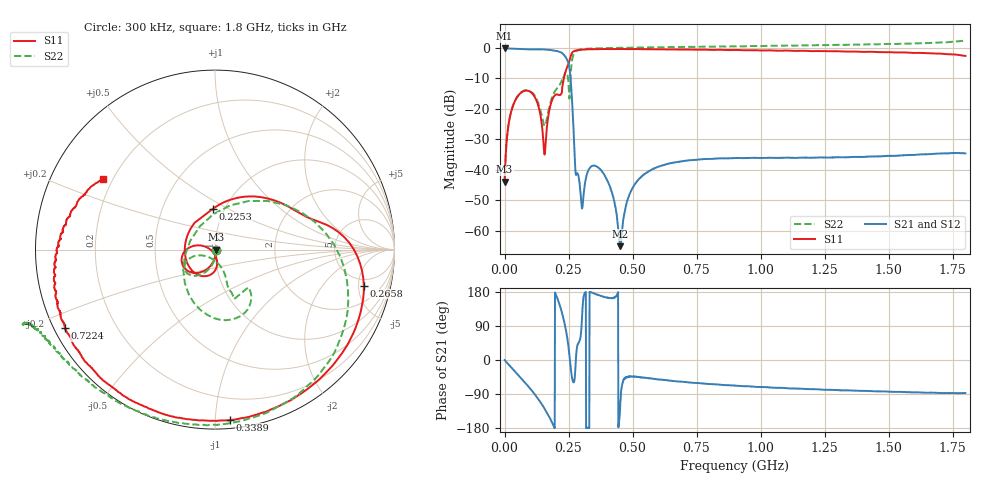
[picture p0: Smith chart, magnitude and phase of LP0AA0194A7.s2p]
!Agilent Technologies,E8358A,US41080443,A.07.50.56
!Agilent E8358A: A.07.50.56
!Date: Wednesday, May 23, 2018 10:03:50
!Correction: S11(Full 2 Port(1,2))
!S21(Full 2 Port(1,2))
!S12(Full 2 Port(1,2))
!S22(Full 2 Port(1,2))
!S2P File: Measurements: S11, S21, S12, S22:
# Hz S  dB  R 50
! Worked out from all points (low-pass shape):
!   1601 points, 300 kHz to 1.8 GHz, reference 50 ohm
!   highest |S21| = -0.11 dB at 300 kHz (marker M1); lowest = -65.0 dB at 451.3 MHz (marker M2)
!   |S21| within 3 dB of the highest: start of sweep to 239.3 MHz
!   lowest |S11| = -43.9 dB at 300 kHz (marker M3), VSWR 1.01, Z = 50.6 - j0.101 ohm
!   |S11| at or under -10 dB: start of sweep to 231.7 MHz
!   |S22| runs from -44.1 to 2.5 dB; largest |S21 - S12| = 0.0093
!   S11 on the Smith chart (normalised r, x): 300 kHz: 1.01, -0.00; 225.3 MHz: 0.88, +0.42; 265.8 MHz: 3.91, -5.78; 338.9 MHz: 0.05, -1.09; 722.4 MHz: 0.03, -0.25; 1.8 GHz: 0.16, +0.28
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300000  -43.86 -8.9  -0.11 -0.2  -0.06 -0.2  -44.08 -9.8
1.8297e7  -23.82 -97.2  -0.19 -13.7  -0.11 -13.7  -23.80 -95.3
4.304288e7  -17.02 -119.6  -0.28 -32.0  -0.21 -32.0  -16.95 -114.5
9.0285e7  -14.05 -157.8  -0.46 -67.6  -0.40 -67.7  -13.84 -144.3
1.296534e8  -18.34 170.1  -0.47 -101.1  -0.40 -101.1  -17.61 -162.3
1.566489e8  -34.98 -132.8  -0.51 -128.6  -0.45 -128.6  -25.58 -117.6
1.971422e8  -15.51 -121.1  -0.90 178.3  -0.84 178.2  -14.19 -70.1
2.252625e8  -12.89 93.4  -1.73 122.5  -1.67 122.5  -11.05 -48.5
2.477588e8  -5.65 22.1  -4.53 45.5  -4.47 45.4  -9.88 -111.2
2.657558e8  -1.38 -13.6  -20.32 -53.2  -20.24 -53.2  -3.09 -3.4
2.792535e8  -0.81 -37.6  -41.68 8.3  -41.62 8.0  -1.05 -43.2
3.006249e8  -0.58 -60.5  -51.49 87.1  -51.57 86.6  -0.47 -69.8
3.388686e8  -0.42 -85.1  -38.85 178.4  -38.81 178.3  -0.18 -93.0
4.063573e8  -0.36 -109.4  -44.36 163.9  -44.30 163.9  -0.02 -113.3
4.513498e8  -0.34 -119.8  -65.03 -128.4  -65.83 -125.8  0.06 -121.6
5.008416e8  -0.37 -128.4  -45.81 -43.6  -45.66 -43.5  0.11 -128.4
6.009499e8  -0.44 -141.7  -38.97 -51.5  -38.90 -51.2  0.22 -138.0
7.224296e8  -0.51 -152.4  -36.87 -59.2  -36.78 -59.6  0.36 -145.3
9.0015e8  -0.66 -162.9  -36.09 -67.4  -36.05 -67.6  0.56 -151.8
1.200475e9  -1.04 -176.2  -36.02 -77.0  -35.96 -77.3  0.85 -157.6
1.5008e9  -1.37 171.9  -35.39 -83.6  -35.38 -83.8  1.31 -158.5
1.8e9  -2.62 147.8  -34.59 -87.0  -34.50 -87.1  2.46 -144.5
